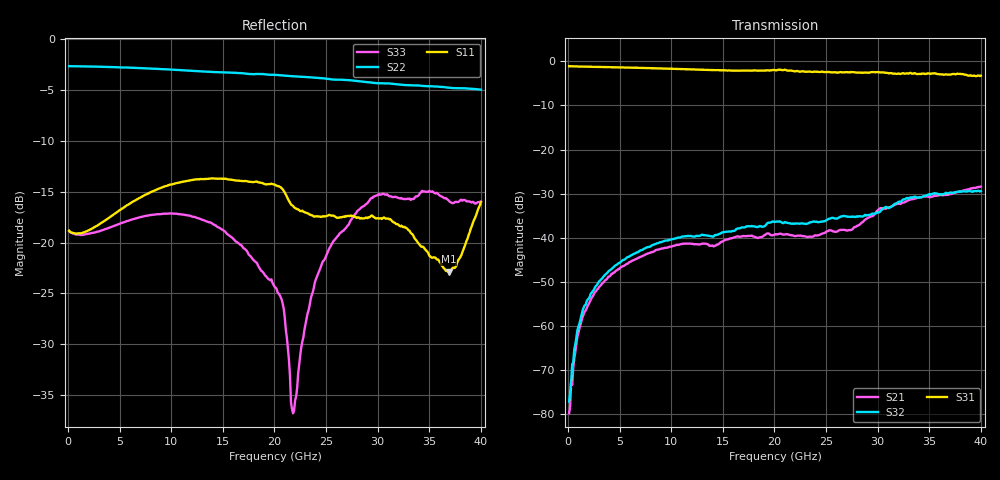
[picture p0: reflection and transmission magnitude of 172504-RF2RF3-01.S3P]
!  3-Port S-parameters saved by WinCal
! VAR MeasName=S-Parameters (CALIBRATED_DATA) read from VNA (N5245A)
! VAR MeasDate=2017-3-15 11:03:58
! VAR NAME=172504-RF2RF3-01
! VAR FILENAME=172504-RF2RF3-01.S3P
! VAR DATE=2017-3-15 11:03:58
! VAR PHYS_PORTS=1,2,3
# Hz S DB R 50
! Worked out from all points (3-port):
!   400 points, 100 MHz to 40 GHz, reference 50 ohm
!   strongest paths, dB at 100 MHz, 10.1 GHz, 20.1 GHz, 30.1 GHz, 40 GHz:
!     S31: -1.1, -1.7, -2.0, -2.5, -3.3
!     S32: -77.1, -40.3, -36.4, -34.2, -29.4
!     S21: -79.7, -41.9, -39.1, -33.5, -28.4
!   lowest |S11| = -22.9 dB at 36.9 GHz (marker M1), VSWR 1.16, Z = 46.7 + j6.17 ohm
!   |S11| at or under -10 dB: start of sweep to end of sweep
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1e8  -18.84 -2.7  -86.39 172.6  -1.10 -0.8
     -79.74 153.0  -2.66 179.8  -89.93 101.0
     -1.10 -0.8  -77.09 81.1  -18.86 -2.4
4e8  -19.03 -8.4  -72.49 97.9  -1.13 -2.8
     -73.26 97.8  -2.67 179.1  -67.72 107.3
     -1.13 -2.8  -68.60 103.0  -19.07 -7.6
1.3e9  -19.08 -22.9  -58.84 95.2  -1.19 -8.3
       -58.78 96.9  -2.68 177.2  -57.35 92.1
       -1.20 -8.4  -57.41 92.4  -19.25 -20.3
4.1e9  -17.47 -59.9  -48.56 69.7  -1.33 -25.3
       -48.56 69.7  -2.75 171.3  -47.13 66.2
       -1.33 -25.2  -47.28 64.6  -18.49 -55.4
1.17e10  -13.90 -116.5  -41.27 18.9  -1.80 -69.8
         -41.29 18.7  -3.09 155.7  -39.52 10.7
         -1.81 -69.6  -39.59 10.4  -17.34 -119.5
2.01e10  -14.35 -150.1  -38.82 -16.7  -2.00 -117.0
         -39.14 -15.0  -3.51 137.7  -36.53 -29.1
         -2.02 -116.9  -36.36 -30.5  -24.42 -146.3
2.18e10  -16.40 -156.0  -39.52 -27.4  -2.37 -129.1
         -39.47 -24.7  -3.65 133.6  -36.84 -37.9
         -2.21 -128.8  -36.75 -39.7  -36.77 -119.4
2.57e10  -17.34 -146.9  -38.55 -34.0  -2.55 -150.4
         -38.54 -32.1  -3.98 123.8  -35.46 -52.6
         -2.46 -150.2  -35.47 -54.2  -19.87 -60.3
3.69e10  -22.86 114.2  -30.15 -107.2  -3.09 139.5
         -30.17 -104.3  -4.77 92.0  -30.22 -122.6
         -3.02 140.0  -29.88 -125.1  -15.89 -94.9
4e10  -16.03 40.2  -28.26 -131.3  -3.28 118.4
      -28.38 -130.5  -4.97 81.5  -29.60 -146.1
      -3.27 118.1  -29.37 -149.8  -15.95 -85.0
